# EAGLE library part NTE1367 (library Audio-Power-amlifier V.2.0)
Dual, Audio Power Amp, 2.3W to 5W (4.6W to 15W BTL)
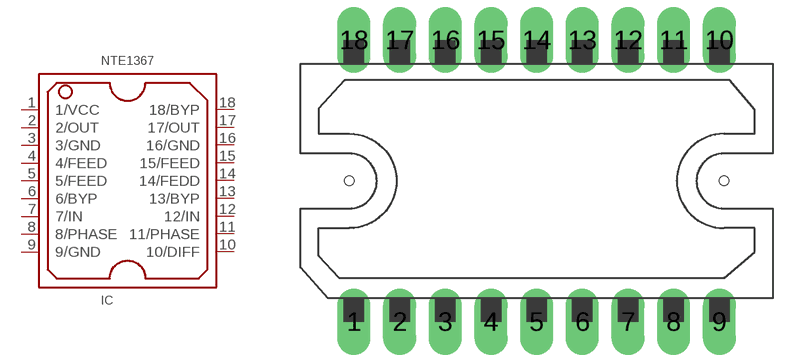
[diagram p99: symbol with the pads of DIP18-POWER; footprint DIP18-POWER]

Designator prefix IC

## NTE1367  [DIP18-POWER]
1  1/VCC  pwr
2  2/OUT  out
3  3/GND  pwr
4  4/FEED
5  5/FEED
6  6/BYP
7  7/IN  in
8  8/PHASE
9  9/GND  pwr
10  10/DIFF
11  11/PHASE
12  12/IN  in
13  13/BYP
14  14/FEDD
15  15/FEED
16  16/GND  pwr
17  17/OUT  out
18  18/BYP

## Footprint DIP18-POWER (pad centres in mm)
drill 1.4 long: 1 -11.6,-8.95; 2 -8.7,-8.95; 3 -5.8,-8.95; 4 -2.9,-8.95; 5 0,-8.95; 6 2.9,-8.95; 7 5.8,-8.95; 8 8.7,-8.95; 9 11.6,-8.95; 10 11.6,8.95; 11 8.7,8.95; 12 5.8,8.95; 13 2.9,8.95; 14 0,8.95; 15 -2.9,8.95; 16 -5.8,8.95; 17 -8.7,8.95; 18 -11.6,8.95
hole 0.6 at -11.9,0
hole 0.6 at 11.9,0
